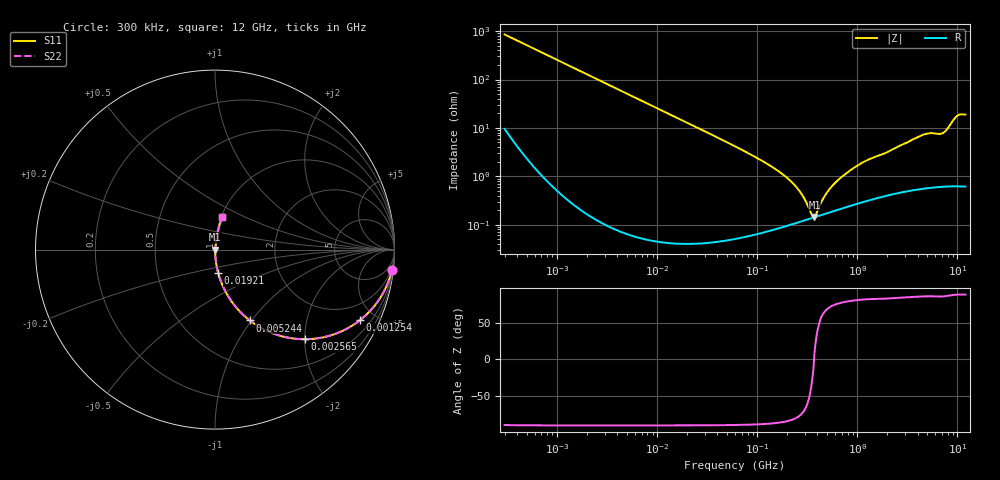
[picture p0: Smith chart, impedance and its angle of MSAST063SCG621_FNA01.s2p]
! MSAST063SCG621_FNA01  S-PARAMETER MODEL  ( General Type )
! Model Generated by TAIYO YUDEN Corporation (http://www.ty-top.com)
! Version 1.0
! TAIYO YUDEN Control No. 160830
! Copyright(c) 2016 TAIYO YUDEN CO.,LTD. All Rights Reserved.
! Product Description (link to TY-COMPAS)
! https://ds.yuden.co.jp/TYCOMPAS/or/detail?pn=MSAST063SCG621JFNA01&u=M
! Products Name : Multilayer Ceramic Capacitors
! Characteristics :
!  Capacitance : 620 pF , Rated Voltage : 25V , TCC : CG / C0G
!  Case Size : 0.6 x 0.3 / 0.024 x 0.012 [mm/inch] , Thickness : 0.3 / 0.012 [mm/inch]
!  (Conditions: Temperature = 25 degC , DC Bias Current/Voltage = 0A / 0V)
! External Node Assignments :
!  1  o---| |---o  2
! GND o---------o GND
! Frequency Range : 0.3MHz  -  12000MHz  [ 401 STEP ]
# MHz S RI R 50
! Freq[MHz].  S11 Real  S11 Imag  S21 Real  S21 Imag  S12 Real  S12 Imag  S22 Real  S22 Imag
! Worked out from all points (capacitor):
!   401 points, 300 kHz to 12 GHz, reference 50 ohm
!   read as one part in series: C = 620 pF near 316.3 kHz
!   lowest |Z| = 144 mohm at 373.3 MHz (marker M1)
!   series resonance near 369.6 MHz, so ESL is about 300 pH
!   S11 on the Smith chart (normalised r, x): 300 kHz: 1, -17; 1.254 MHz: 1.01, -4.09; 2.565 MHz: 1.00, -2.00; 5.244 MHz: 1.00, -0.98; 19.21 MHz: 1.00, -0.27; 12 GHz: 1.01, +0.38
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0.3  0.9853 -0.115  0.0147 0.115  0.0147 0.115  0.9853 -0.115
0.681995  0.9334 -0.2478  0.0666 0.2478  0.0666 0.2478  0.9334 -0.2478
1.254294  0.8069 -0.3939  0.1931 0.3939  0.1931 0.3939  0.8069 -0.3939
1.769972  0.6775 -0.4667  0.3225 0.4667  0.3225 0.4667  0.6775 -0.4667
2.564711  0.5004 -0.4994  0.4996 0.4994  0.4996 0.4994  0.5004 -0.4994
5.244178  0.1935 -0.3944  0.8065 0.3944  0.8065 0.3944  0.1935 -0.3944
10.44266  0.0573 -0.2315  0.9427 0.2315  0.9427 0.2315  0.0573 -0.2315
19.20568  0.0178 -0.1309  0.9822 0.1309  0.9822 0.1309  0.0178 -0.1309
60  0.00224 -0.0416  0.9978 0.0416  0.9978 0.0416  0.00224 -0.0416
125.9782  0.00105 -0.018  0.999 0.018  0.999 0.018  0.00105 -0.018
202.9496  0.00104 -0.00889  0.999 0.00889  0.999 0.00889  0.00104 -0.00889
271.6094  0.00117 -0.00444  0.9988 0.00444  0.9988 0.00444  0.00117 -0.00444
353.9943  0.00137 -0.000727  0.9986 0.000727  0.9986 0.000727  0.00137 -0.000727
373.2558  0.00142 0.000219  0.9986 -0.000219  0.9986 -0.000219  0.00142 0.000219
499.5319  0.00174 0.00434  0.9983 -0.00434  0.9983 -0.00434  0.00174 0.00434
668.5285  0.00217 0.00874  0.9978 -0.00874  0.9978 -0.00874  0.00217 0.00874
1135.593  0.00328 0.0191  0.9967 -0.0191  0.9967 -0.0191  0.00328 0.0191
2088.533  0.00515 0.0326  0.9949 -0.0326  0.9949 -0.0326  0.00515 0.0326
4623.766  0.0108 0.072  0.9892 -0.072  0.9892 -0.072  0.0108 0.072
7064.448  0.0118 0.0758  0.9882 -0.0758  0.9882 -0.0758  0.0118 0.0758
9968.853  0.0365 0.171  0.9635 -0.171  0.9635 -0.171  0.0365 0.171
12000  0.04 0.1805  0.96 -0.1805  0.96 -0.1805  0.04 0.1805
